(* 	
	Program Name: 	ACS_CMD_ENABLE
	Purpose:		Copy Enable Command to ACS Drive Output Command Register
	When Executed:	Enables drive and clears safety faults (critical faults cannot be cleared)
*)
PROGRAM ACS_CMD_ENABLE
VAR_IN_OUT
	Axis:ACS_DRIVE_TYPE;
END_VAR
VAR
	_command:	USINT	:= ACS_COMMANDS.ENABLE;
END_VAR

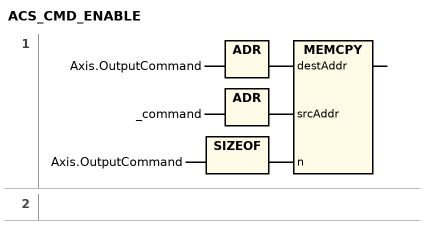
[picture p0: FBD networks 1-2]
// NETWORK 1
MEMCPY(destAddr := ADR(Axis.OutputCommand), srcAddr := ADR(_command), n := SIZEOF(Axis.OutputCommand));

// NETWORK 2

END_PROGRAM
